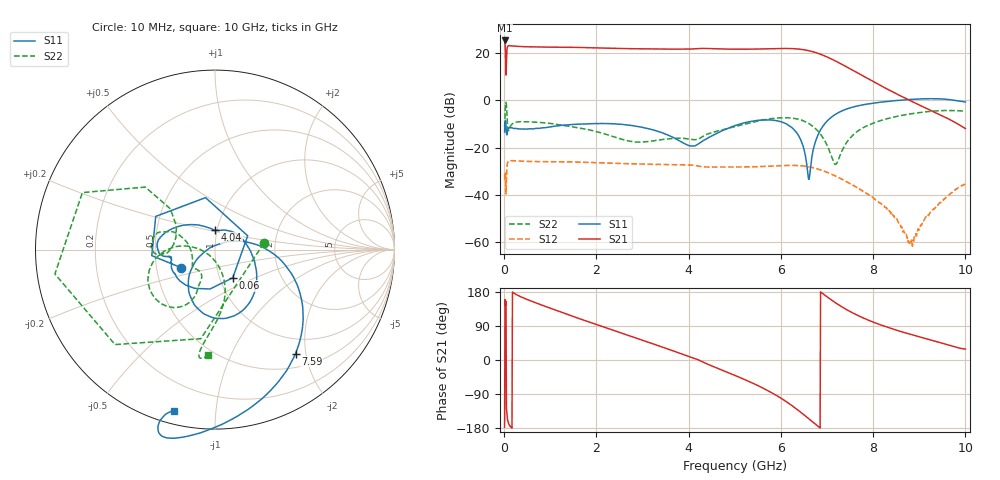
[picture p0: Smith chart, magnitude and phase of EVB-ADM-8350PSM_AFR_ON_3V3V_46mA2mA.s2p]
!Keysight Technologies,N5247B,US58420632,A.15.75.19
!Date: Monday, January 30, 2023 13:25:24
!Correction: S11(C  2-Port  )
!S21(C  2-Port  )
!S12(C  2-Port  )
!S22(C  2-Port  )
!S2P File: Measurements: S11, S21, S12, S22:
# Hz S  dB  R 50
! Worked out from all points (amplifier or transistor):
!   1000 points, 10 MHz to 10 GHz, reference 50 ohm
!   highest |S21| = 25.3 dB at 10 MHz (marker M1)
!   |S21| within 3 dB of that: 68.56 MHz to 1.716 GHz (1.648 GHz wide, 185 % of centre)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
!   unconditionally stable (mu >= 1): start of sweep to 867 MHz; 2.472 GHz to 5.319 GHz; 6.331 GHz to 8.522 GHz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
!   at 1.67 GHz: K = 0.96, MSG = 24.2 dB, |S12| = -26.1 dB
!   at 5.01 GHz: K = 1.09, MAG = 23.1 dB, |S12| = -28.2 dB
!   at 10 GHz: K = 10.41, MAG = -1.4 dB, |S12| = -35.4 dB
!   S11 on the Smith chart (normalised r, x): 10 MHz: 0.67, -0.14; 60 MHz: 1.15, -0.38; 4.04 GHz: 0.98, +0.22; 7.59 GHz: 0.72, -1.81; 10 GHz: 0.06, -0.78
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1e7  -13.35 -152.2  25.27 -177.3  -33.66 74.7  -11.24 7.4
6e7  -14.62 -57.8  21.20 -141.9  -28.06 65.6  -5.65 138.1
8e7  -12.26 -117.6  22.87 -160.4  -26.06 41.2  -12.00 148.8
1e8  -11.64 -137.8  23.06 -168.6  -25.61 29.4  -12.66 173.0
1.4e8  -11.56 -152.4  23.03 -176.1  -25.50 17.8  -10.81 -175.4
3.2e8  -12.08 -166.2  22.76 169.2  -25.61 -1.5  -9.07 179.3
1.02e9  -11.18 -172.0  22.46 135.7  -25.90 -30.0  -9.81 162.4
1.68e9  -10.02 -178.3  22.29 107.0  -26.14 -51.9  -11.86 157.1
2.46e9  -10.06 168.5  21.91 74.4  -26.63 -76.3  -15.91 166.0
3.34e9  -13.11 142.0  21.66 37.9  -27.07 -105.1  -16.82 -150.4
4.04e9  -19.24 89.0  21.64 8.2  -27.34 -131.6  -16.42 -134.3
4.4e9  -16.10 26.8  21.88 -10.4  -28.17 -143.8  -14.30 -114.2
5.01e9  -10.62 -38.0  21.58 -41.0  -28.19 -164.3  -11.09 -113.5
5.6e9  -8.30 -75.0  21.70 -73.5  -27.95 171.5  -8.38 -122.6
6e9  -9.04 -103.1  21.88 -100.7  -27.61 150.6  -7.38 -137.7
6.31e9  -12.92 -131.0  21.76 -126.7  -27.49 130.0  -7.67 -154.5
6.67e9  -24.10 38.3  20.64 -161.6  -28.31 101.9  -10.67 -176.9
7.09e9  -7.19 -16.5  17.50 158.7  -31.13 70.8  -23.29 -174.4
7.59e9  -2.70 -52.3  12.33 122.2  -36.15 43.3  -14.18 -74.0
8.34e9  -0.39 -85.2  4.39 85.2  -46.45 26.4  -7.59 -90.2
8.83e9  0.39 -97.7  -0.38 67.0  -60.00 106.1  -5.64 -96.8
1e10  -0.68 -104.1  -11.91 28.8  -35.37 113.3  -4.60 -93.7
